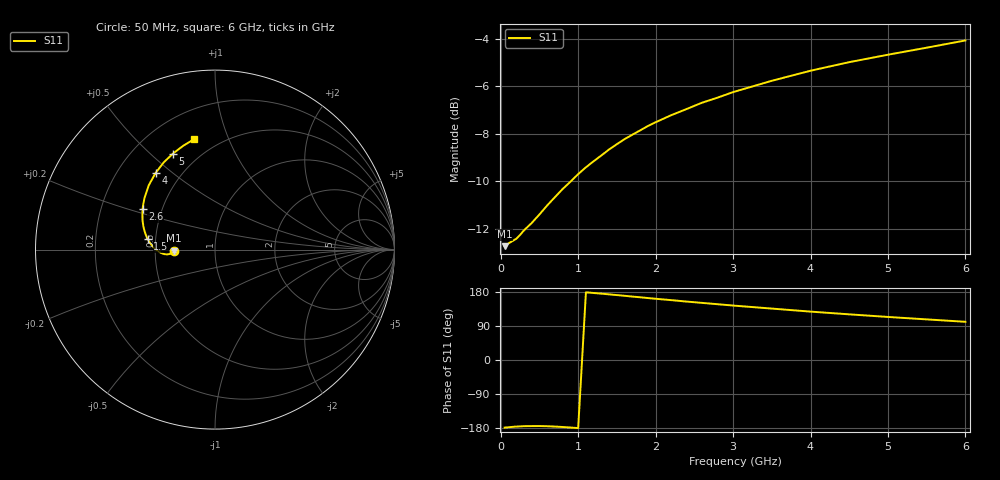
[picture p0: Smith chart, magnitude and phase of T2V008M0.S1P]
! SIEMENS Discrete & RF Semiconductors
! BAS70-04W
! Si Schottky Diode in SOT323
! IF = 8 mA
! S-Parameters:  November  1997
# GHz  S  MA  R  50
!  f  S11
! GHz  MAG  ANG
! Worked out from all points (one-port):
!   34 points, 50 MHz to 6 GHz, reference 50 ohm
!   lowest |S11| = -12.7 dB at 50 MHz (marker M1), VSWR 1.60, Z = 31.2 - j0.425 ohm
!   |S11| at or under -10 dB: start of sweep to 906 MHz
!   S11 on the Smith chart (normalised r, x): 50 MHz: 0.62, -0.01; 1.5 GHz: 0.45, +0.06; 2.6 GHz: 0.39, +0.22; 4 GHz: 0.36, +0.44; 5 GHz: 0.36, +0.59; 6 GHz: 0.37, +0.76
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0.05  0.2308 -178.4
0.2  0.2392 -175.7
0.25  0.2438 -175.3
0.3  0.2493 -174.6
0.4  0.2583 -174.4
0.5  0.2692 -174.3
0.6  0.2813 -174.8
0.7  0.2928 -175.7
0.8  0.3047 -176.8
1  0.3274 -179.7
1.1  0.3384 178.6
1.3  0.3585 175.1
1.4  0.369 173.2
1.5  0.3786 171.3
1.6  0.388 169.4
1.8  0.4047 165.5
1.9  0.4134 163.5
2  0.421 161.6
2.2  0.4356 158.0
2.4  0.4489 154.2
2.6  0.4629 150.7
3  0.4873 143.7
3.5  0.5148 135.7
4  0.5405 127.7
4.5  0.5635 120.5
5  0.5842 113.6
5.5  0.6045 107.2
6  0.626 100.8
